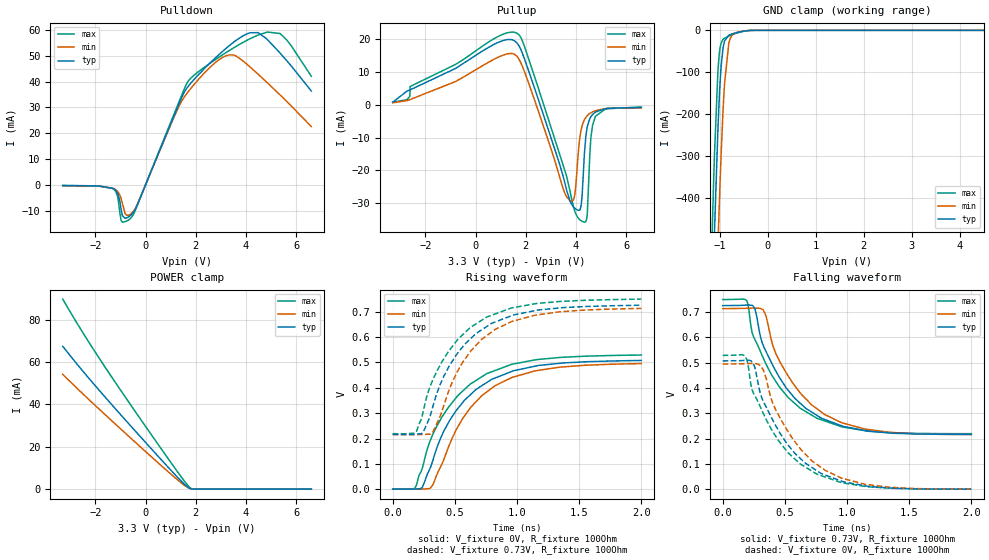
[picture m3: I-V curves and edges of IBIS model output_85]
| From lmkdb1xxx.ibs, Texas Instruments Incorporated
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[Model]   output_85
Model_type   Output
Polarity   Non-Inverting
Vmeas = 0.365
Vref = 0
Cref = 2pF
Rref = 100000
|   typ   min   max
C_comp   5pF   4.5pF   5.5pF
[Voltage Range]   3.3   3.135   3.465
[Temperature Range]   27   125   -40
[Pullup Reference]   3.3   3.135   3.465
[Pulldown Reference]   0   -0   0
[Power Clamp Reference]   3.3   3.135   3.465
[GND Clamp Reference]   0   0   0
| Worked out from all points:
|   slope of the pulldown table from 0 to 0.495 V, typ, clamps not added: 42.1 ohm
|   GND clamp passes 1 mA (typ) near -0.44 V on its own axis
|   falling waveform, V_fixture 0.73V, R_fixture 100Ohm: 20-80 % time 377ps typ, 384ps min, 383ps max; typ from 0.725 V to 0.217 V
|   rising waveform, V_fixture 0V, R_fixture 100Ohm: 20-80 % time 396ps typ, 395ps min, 402ps max; typ from 0.001 V to 0.508 V
|   rising waveform, V_fixture 0.73V, R_fixture 100Ohm: 20-80 % time 382ps typ, 377ps min, 390ps max; typ from 0.217 V to 0.725 V
|   falling waveform, V_fixture 0V, R_fixture 100Ohm: 20-80 % time 378ps typ, 384ps min, 386ps max; typ from 0.507 V to 0.001 V
[Pulldown]
|   Voltage   I(typ)   I(min)   I(max)
-3.3V     -318.6uA   -393.1uA   -273.4uA
-1.31V    -1.398mA   -1.371mA   -1.435mA
-1.122V   -3.194mA   -2.494mA   -4.283mA
-973.5mV  -9.578mA   -5.349mA   -13.87mA
-815.1mV  -13.03mA   -11.21mA   -14.32mA
-636.9mV  -12.23mA   -11.62mA   -13.37mA
-379.5mV  -8.892mA   -8.671mA   -9.227mA
1.68V     37.96mA    35.85mA    39.95mA
3.244V    53.25mA    50.17mA    51.53mA
4.481V    59.02mA    42.89mA    58.09mA
5.353V    51.13mA    34.87mA    58.68mA
6.6V      36.35mA    22.57mA    42.09mA
[GND Clamp]
|   Voltage   I(typ)   I(min)   I(max)
-3.3V     -10.93A    -11.17A    -10.79A
-1.211V   -881.9mA   -1.2A      -686.4mA
-1.132V   -556.2mA   -867.4mA   -367.4mA
-1.112V   -480.1mA   -787.6mA   -296.1mA
-1.033V   -214.5mA   -487.9mA   -84.47mA
-1.013V   -162.9mA   -419.7mA   -57.48mA
-973.5mV  -85.09mA   -295mA     -30.33mA
-904.2mV  -25.82mA   -129mA     -18.86mA
-815.1mV  -11.68mA   -31.98mA   -13.66mA
-785.4mV  -10.14mA   -20.14mA   -12.18mA
-320.1mV  -99.39uA   -119.7uA   -85.22uA
6.6V      0A         0A         0A
[Pullup]
|   Voltage   I(typ)   I(min)   I(max)
-3.3V     815.4uA    650uA      792.1uA
848.1mV   18.92mA    14.39mA    20.72mA
1.65V     18.91mA    14.82mA    21.89mA
3.759V    -29.34mA   -29.32mA   -26.28mA
3.957V    -31.62mA   -27.07mA   -32.62mA
4.165V    -31.9mA    -9.367mA   -35.19mA
4.234V    -28.48mA   -6.653mA   -35.54mA
4.333V    -14.99mA   -4.554mA   -35.85mA
4.452V    -6.575mA   -3.241mA   -32.96mA
4.6V      -3.505mA   -2.356mA   -9.462mA
4.769V    -2.234mA   -1.788mA   -3.599mA
6.6V      -765.3uA   -936uA     -660uA
[POWER Clamp]
|   Voltage   I(typ)   I(min)   I(max)
-3.3V     67.46mA    54.22mA    89.73mA
-2.28V    52.65mA    42.55mA    69.77mA
-1.221V   38.21mA    30.92mA    50.67mA
1.175V    6.833mA    5.39mA     9.808mA
1.601V    1.727mA    1.368mA    2.963mA
1.789V    238.8uA    261.4uA    521.2uA
1.977V    4.57uA     9.613uA    7.6uA
6.6V      0A         0A         0A
[Ramp]
R_load = 100
|   typ   min   max
dV/dt_r   0.303987/3.95814e-10   0.296571/3.95271e-10   0.316807/4.01973e-10
dV/dt_f   0.304714/3.77209e-10   0.297744/3.83928e-10   0.317433/3.83478e-10
[Falling Waveform]
V_fixture = 0.73V
V_fixture_min = 0.72V
V_fixture_max = 0.75V
R_fixture = 100Ohm
C_fixture = 0F
|   Time   V(typ)   V(min)   V(max)
0s        725.2mV    713.2mV    749.2mV
190.9ps   727.4mV    714.7mV    745.7mV
237.4ps   726.4mV    715.4mV    617.5mV
258.9ps   714mV      715.5mV    591.4mV
326.6ps   567.8mV    708.4mV    518.1mV
449.8ps   447.3mV    513.6mV    409.1mV
629.2ps   337.7mV    377.4mV    318.8mV
757.1ps   292.6mV    318.7mV    281.1mV
1.146ns   232.2mV    238.1mV    231.9mV
2ns       217.4mV    217mV      220.1mV
[Rising Waveform]
V_fixture = 0V
V_fixture_min = 0V
V_fixture_max = 0V
R_fixture = 100Ohm
C_fixture = 0F
|   Time   V(typ)   V(min)   V(max)
0s        1.066mV    1.044mV    1.166mV
178.4ps   1.408mV    1.066mV    4.711mV
240.1ps   9.264mV    1.576mV    86.72mV
304.2ps   87.01mV    5.2mV      194.8mV
378.6ps   194.2mV    82.33mV    269.7mV
511.2ps   311.2mV    235.5mV    361.9mV
629.2ps   374.8mV    324.2mV    416.3mV
757.1ps   421mV      384mV      456mV
1.146ns   485.3mV    467mV      510mV
2ns       507.7mV    495.3mV    529.2mV
[Rising Waveform]
V_fixture = 0.73V
V_fixture_min = 0.72V
V_fixture_max = 0.75V
R_fixture = 100Ohm
C_fixture = 0F
|   Time   V(typ)   V(min)   V(max)
0s        216.6mV    215.6mV    219.4mV
190.9ps   217.8mV    215.7mV    228.2mV
240.1ps   221.8mV    216.5mV    295.6mV
326.6ps   332.2mV    228.7mV    435.9mV
413.4ps   447.6mV    333.3mV    516mV
513ps     530.4mV    457.8mV    584.1mV
629.2ps   594.8mV    546.1mV    639mV
757.1ps   641.5mV    605.9mV    678.9mV
1.146ns   704.1mV    686.1mV    731.2mV
2ns       725.2mV    712.8mV    749.5mV
[Falling Waveform]
|Gnd
V_fixture = 0V
V_fixture_min = 0V
V_fixture_max = 0V
R_fixture = 100Ohm
C_fixture = 0F
|   Time   V(typ)   V(min)   V(max)
0s        507.2mV    494.8mV    528.9mV
178.4ps   509.4mV    496.3mV    526.1mV
201.1ps   510.2mV    496.7mV    499.3mV
240.1ps   501.9mV    497.4mV    388.6mV
304.2ps   376.3mV    487.8mV    324.1mV
402.5ps   273.8mV    340.3mV    228.2mV
475.7ps   211.1mV    269.6mV    176mV
757.1ps   74.24mV    98.95mV    60.57mV
1.146ns   14.41mV    20.39mV    11.9mV
2ns       1.212mV    1.363mV    1.222mV
